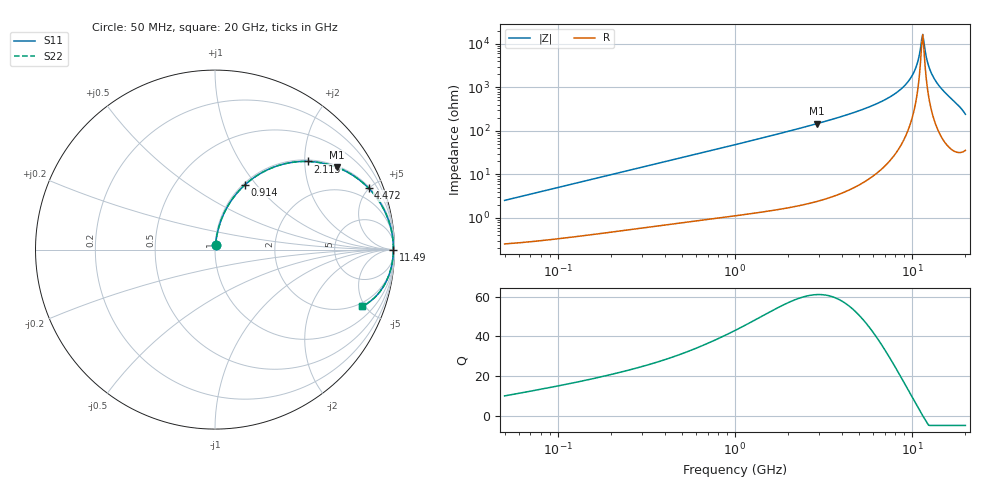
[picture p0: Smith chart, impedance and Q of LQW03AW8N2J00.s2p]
!Murata Part Number: LQW03AW8N2J00
!These Parameters are Measured in Series Mode Connection
!  o--[Z]--o
!Port1  Port2
!  o-------o
!Freq. Start=50[MHz] Stop=20[GHz], 401[Steps]
# Hz S RI R 50
!Freq.(Hz) S11(Real) S11(Imag) S21(Real) S21(Imag) S12(Real) S12(Imag) S22(Real) S22(Imag)
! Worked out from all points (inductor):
!   401 points, 50 MHz to 20 GHz, reference 50 ohm
!   read as one part in series: L = 8 nH near 51.52 MHz
!   highest Q = 61.2 at 2.896 GHz (marker M1), where L = 8.03 nH
!   self-resonance near 11.32 GHz
!   S11 on the Smith chart (normalised r, x): 50 MHz: 1.01, +0.05; 914 MHz: 1.02, +0.88; 2.115 GHz: 1.04, +2.08; 4.472 GHz: 1.09, +4.95; 11.49 GHz: open; 20 GHz: 1.71, -4.77
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5e7  0.00316 0.0251  0.9968 -0.0251  0.9968 -0.0251  0.00316 0.0251
1.364002e8  0.00834 0.0667  0.9917 -0.0667  0.9917 -0.0667  0.00834 0.0667
3.721004e8  0.0376 0.1727  0.9624 -0.1727  0.9624 -0.1727  0.0376 0.1727
9.140482e8  0.1682 0.3621  0.8318 -0.3621  0.8318 -0.3621  0.1682 0.3621
1e9  0.1938 0.3838  0.8062 -0.3838  0.8062 -0.3838  0.1938 0.3838
2.114743e9  0.5184 0.4911  0.4816 -0.4911  0.4816 -0.4911  0.5184 0.4911
2.728004e9  0.6493 0.4691  0.3507 -0.4691  0.3507 -0.4691  0.6493 0.4691
2.896447e9  0.6786 0.4589  0.3214 -0.4589  0.3214 -0.4589  0.6786 0.4589
4.472136e9  0.8552 0.3429  0.1448 -0.3429  0.1448 -0.3429  0.8552 0.3429
7.442007e9  0.967 0.1625  0.033 -0.1625  0.033 -0.1625  0.967 0.1625
8.774992e9  0.9839 0.1018  0.0161 -0.1018  0.0161 -0.1018  0.9839 0.1018
9.892087e9  0.991 0.057  0.00895 -0.057  0.00895 -0.057  0.991 0.057
1.050288e10  0.993 0.0343  0.00695 -0.0343  0.00695 -0.0343  0.993 0.0343
1.082228e10  0.9936 0.0227  0.00636 -0.0227  0.00636 -0.0227  0.9936 0.0227
1.115139e10  0.9939 0.0111  0.00605 -0.0111  0.00605 -0.0111  0.9939 0.0111
1.149051e10  0.994 -0.000604  0.00603 0.000604  0.00603 0.000604  0.994 -0.000604
1.166392e10  0.9939 -0.00653  0.00613 0.00653  0.00613 0.00653  0.9939 -0.00653
1.220001e10  0.9931 -0.0245  0.00691 0.0245  0.00691 0.0245  0.9931 -0.0245
1.257102e10  0.9922 -0.0368  0.00785 0.0368  0.00785 0.0368  0.9922 -0.0368
1.354865e10  0.9881 -0.0685  0.0119 0.0685  0.0119 0.0685  0.9881 -0.0685
1.747767e10  0.941 -0.2017  0.059 0.2017  0.059 0.2017  0.941 -0.2017
2e10  0.8196 -0.3168  0.1804 0.3168  0.1804 0.3168  0.8196 -0.3168
